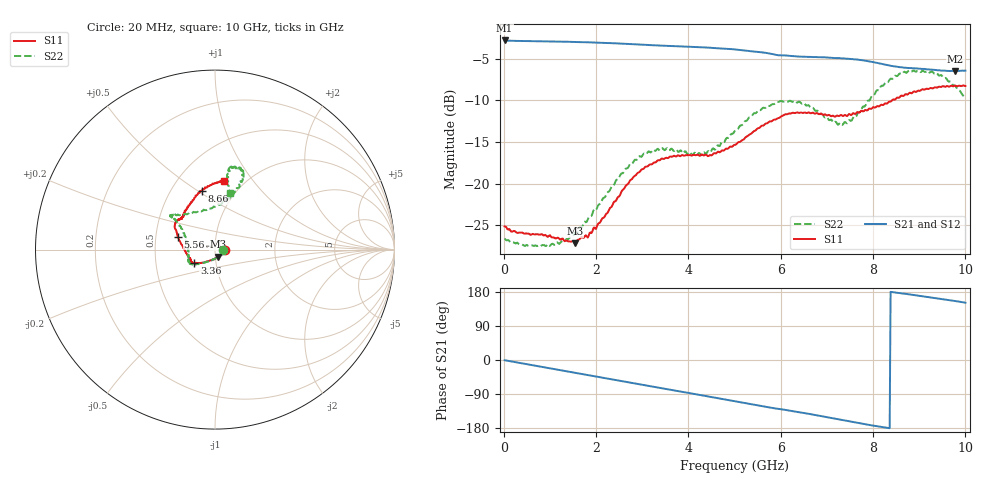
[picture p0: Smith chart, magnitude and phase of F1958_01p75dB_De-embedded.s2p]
! Integrated Device Technology
! Corporate Headquarters
! 6024 Silver Creek Valley Road
! San Jose, CA 95138  USA
! Phone:  1-408-284-8200
! Toll Free:  1-800-223-1366
! Webpage:  http://www.idt.com/
! Timing and RF Division
! 515 Groton Road, Suite 102
! Westford, MA 01886-6024
! Device:  F1958
! Description: 7-bit 0.25 dB Digital Step Attenuator
! Frequency:  0.001 -  6.000 GHz
! Package:  4x4 mm Thin QFN Plastic Package: 24 pin
! Ports:  2 RF, 12 DC
!  Pin  1  = D0
!  Pin  2  = VDD
!  Pin  3  = VMODE
!  Pin  4  = GND
!  Pin  5  = RF1  =  Port 1
!  Pin  6  = GND
!  Pin  7  = GND
!  Pin  8  = GND
!  Pin  9  = GND
!  Pin 10  = GND
!  Pin 11  = GND
!  Pin 12  = GND
!  Pin 13  = GND
!  Pin 14  = RF2  =  Port 2
!  Pin 15  = GND
!  Pin 16  = LE
!  Pin 17  = CLK
!  Pin 18  = DATA
!  Pin 19  = D6
!  Pin 20  = D5
!  Pin 21  = D4
!  Pin 22  = D3
!  Pin 23  = D2
!  Pin 24  = D1
! State:  7
! Atten State:  1.75 dB
! Voltage:  +3.30 Volts
! Current:  0.258 mA
! Data:  The device was measured on a F1958 evaluation board which has
!  individual transmission lines to the RF pins.  Data was collected
!  using a calibrated network analyzer.  The evaluation board was
!  de-embedded using Automatic Fixture Removal (AFR).
!  The reference plane is the edge of the package pin.
! Misc:
!  Action Tracker AT0419
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# GHz S dB R 50
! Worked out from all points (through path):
!   500 points, 20 MHz to 10 GHz, reference 50 ohm
!   highest |S21| = -2.81 dB at 20 MHz (marker M1); lowest = -6.5 dB at 9.78 GHz (marker M2)
!   group delay of S21, straight-line fit = 58.8 ps
!   lowest |S11| = -27.2 dB at 1.54 GHz (marker M3), VSWR 1.09, Z = 51.8 - j4.08 ohm
!   |S11| at or under -10 dB: start of sweep to 8.413 GHz
!   |S22| runs from -27.5 to -6.4 dB; largest |S21 - S12| = 0.0019
!   S11 on the Smith chart (normalised r, x): 20 MHz: 1.12, -0.01; 3.36 GHz: 0.79, -0.12; 5.56 GHz: 0.65, +0.10; 8.66 GHz: 0.70, +0.52; 10 GHz: 0.81, +0.73
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0.02  -25.15 -2.4  -2.81 -0.6  -2.82 -0.6  -26.59 -3.3
0.44  -26.01 -9.4  -2.88 -9.7  -2.88 -9.7  -27.45 -17.3
0.96  -26.41 -27.7  -2.92 -21.0  -2.92 -21.0  -27.28 -43.9
1.54  -27.17 -63.7  -3.00 -33.6  -2.99 -33.6  -25.95 -87.8
1.7  -26.45 -75.5  -3.02 -37.0  -3.02 -37.0  -25.23 -99.3
2.02  -25.13 -101.3  -3.08 -44.1  -3.07 -44.0  -22.97 -117.5
2.72  -19.80 -134.5  -3.24 -59.3  -3.23 -59.3  -17.82 -141.3
3.04  -18.17 -142.5  -3.33 -66.3  -3.32 -66.4  -16.39 -146.7
3.36  -17.21 -146.7  -3.42 -73.2  -3.43 -73.3  -15.94 -151.2
4.32  -16.61 -157.9  -3.64 -93.8  -3.65 -93.8  -16.28 177.2
5.02  -15.34 179.7  -3.90 -109.2  -3.91 -109.2  -13.56 149.9
5.56  -13.19 160.6  -4.23 -120.9  -4.24 -120.9  -11.19 143.3
6.02  -11.90 151.8  -4.60 -130.1  -4.61 -130.1  -10.10 142.7
6.68  -11.50 141.6  -4.80 -143.5  -4.82 -143.4  -10.91 136.6
7.2  -11.90 136.7  -4.93 -155.0  -4.94 -154.8  -12.62 112.7
7.4  -11.76 134.8  -5.00 -159.5  -5.00 -159.4  -12.62 98.5
7.92  -10.98 123.4  -5.33 -171.4  -5.33 -171.4  -10.03 73.3
8.34  -10.19 112.0  -5.81 -179.7  -5.81 -179.7  -7.70 68.3
8.66  -9.49 102.6  -6.08 175.3  -6.08 175.3  -6.64 70.2
9.28  -8.57 88.4  -6.33 164.3  -6.34 164.3  -6.53 79.0
9.78  -8.23 82.9  -6.49 155.6  -6.52 155.6  -8.25 79.2
10  -8.28 82.5  -6.43 151.1  -6.46 151.2  -9.76 74.8
